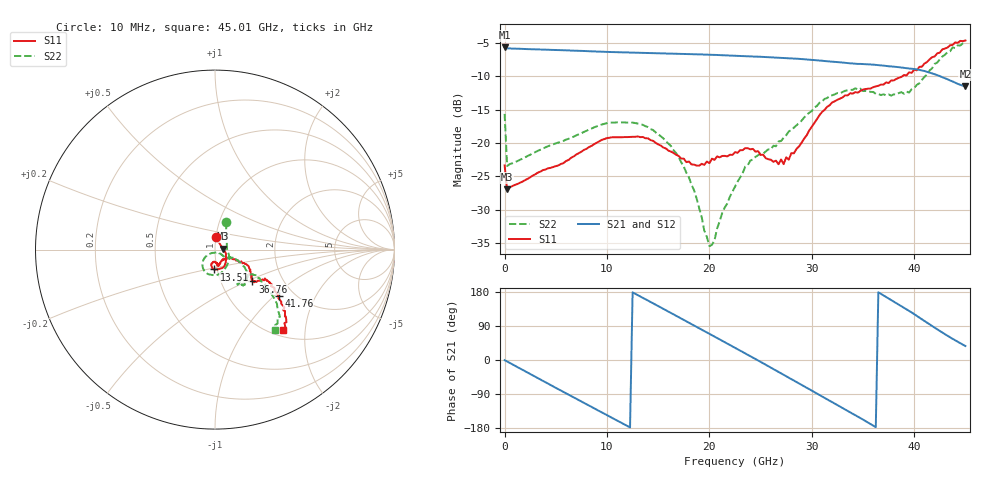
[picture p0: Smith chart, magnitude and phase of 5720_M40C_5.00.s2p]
! Device:  ADRF5720
! Description: 0.5dB LSB GaAs MMIC 6-bit Digital Attenuator
! Frequency:  0.000009 -  40 GHz
! Ports:
!	RF1	= Port 1
!	RF2	= Port 2
! Vdd:  3.3 Volt
! Vss:  -3.3 Volt
! Control:  0/3.3 Volt
! State:  5.00 dB attenuation
! Data:  The device was measured using G-S-G Probes on a matrix board.
!  Data was collected using an calibrated 4 port network analyzer.
!  The reference plane for this measurement is at the launchers.
! Note:  Analog Devices supplies this data as a sample of measured data
!  for this product.  Your particular data for this product may vary.
!  Data was taken at -40 degrees C.
!  Analog Devices reserves the right to change this data at anytime.
# GHZ S DB R 45.0
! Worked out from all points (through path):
!   181 points, 10 MHz to 45.01 GHz, reference 45 ohm
!   highest |S21| = -5.66 dB at 10 MHz (marker M1); lowest = -11.5 dB at 45.01 GHz (marker M2)
!   group delay of S21, straight-line fit = 41.8 ps
!   lowest |S11| = -27.0 dB at 260 MHz (marker M3), VSWR 1.09, Z = 49.2 + j0.536 ohm
!   |S11| at or under -10 dB: start of sweep to 38.85 GHz
!   |S22| runs from -35.5 to -5.0 dB; largest |S21 - S12| = 0.002
!   S11 on the Smith chart (normalised r, x): 10 MHz: 1.00, +0.14; 13.51 GHz: 0.96, -0.22; 36.76 GHz: 1.41, -0.54; 41.76 GHz: 1.66, -1.07; 45.01 GHz: 1.12, -1.53
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0.01  -23.38 87.2  -5.66 -0.4  -5.68 -0.4  -15.65 68.4
0.26  -26.99 7.0  -5.82 -4.0  -5.83 -4.1  -23.47 3.2
2.01  -25.59 -8.7  -5.91 -29.8  -5.93 -29.9  -22.16 -15.4
4.26  -23.81 -18.9  -6.03 -62.6  -6.05 -62.6  -20.49 -32.5
6.01  -22.72 -32.8  -6.11 -88.0  -6.13 -88.0  -19.51 -47.6
7.76  -21.05 -46.3  -6.21 -113.2  -6.23 -113.3  -18.35 -63.3
10.76  -19.15 -69.6  -6.38 -156.4  -6.40 -156.4  -16.95 -89.4
13.51  -19.12 -93.0  -6.50 164.1  -6.51 164.0  -17.29 -114.3
15.26  -20.40 -101.5  -6.55 138.7  -6.57 138.6  -19.00 -128.7
18.01  -22.79 -99.0  -6.67 98.5  -6.69 98.5  -25.18 -145.5
20.01  -23.04 -86.5  -6.77 69.1  -6.79 69.0  -35.50 -94.3
20.51  -22.55 -84.0  -6.80 61.7  -6.82 61.6  -34.61 -54.3
22.76  -21.48 -81.3  -6.94 28.5  -6.96 28.4  -25.83 -36.4
25.01  -21.81 -71.5  -7.08 -4.9  -7.10 -5.1  -21.59 -33.1
27.26  -23.19 -49.5  -7.26 -38.8  -7.27 -39.0  -19.22 -24.4
30.26  -17.00 -25.1  -7.56 -84.7  -7.59 -84.8  -14.69 -30.4
33.76  -12.55 -32.0  -8.06 -138.1  -8.09 -138.3  -12.05 -47.5
36.76  -11.25 -40.4  -8.37 174.6  -8.39 174.4  -12.83 -57.2
37.76  -10.64 -37.9  -8.53 158.4  -8.56 158.2  -12.91 -53.3
39.51  -9.41 -30.9  -8.84 129.6  -8.86 129.5  -12.46 -35.8
41.76  -7.15 -36.3  -9.57 89.8  -9.59 89.5  -8.80 -36.4
45.01  -4.63 -49.6  -11.52 36.9  -11.55 36.7  -5.04 -53.1
